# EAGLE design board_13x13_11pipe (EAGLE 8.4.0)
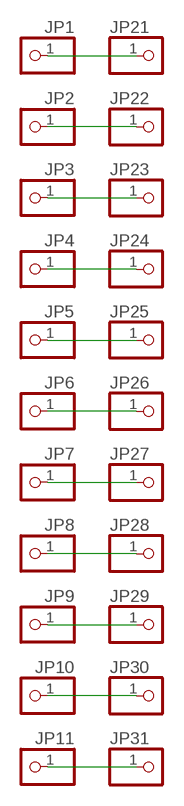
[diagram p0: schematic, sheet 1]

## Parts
JP1  PINHD-1X1CB  [1X01-CLEANBIG]
JP2  PINHD-1X1CB  [1X01-CLEANBIG]
JP3  PINHD-1X1CB  [1X01-CLEANBIG]
JP4  PINHD-1X1CB  [1X01-CLEANBIG]
JP5  PINHD-1X1CB  [1X01-CLEANBIG]
JP6  PINHD-1X1CB  [1X01-CLEANBIG]
JP7  PINHD-1X1CB  [1X01-CLEANBIG]
JP8  PINHD-1X1CB  [1X01-CLEANBIG]
JP9  PINHD-1X1CB  [1X01-CLEANBIG]
JP10  PINHD-1X1CB  [1X01-CLEANBIG]
JP11  PINHD-1X1CB  [1X01-CLEANBIG]
JP21  PINHD-1X1CB  [1X01-CLEANBIG]
JP22  PINHD-1X1CB  [1X01-CLEANBIG]
JP23  PINHD-1X1CB  [1X01-CLEANBIG]
JP24  PINHD-1X1CB  [1X01-CLEANBIG]
JP25  PINHD-1X1CB  [1X01-CLEANBIG]
JP26  PINHD-1X1CB  [1X01-CLEANBIG]
JP27  PINHD-1X1CB  [1X01-CLEANBIG]
JP28  PINHD-1X1CB  [1X01-CLEANBIG]
JP29  PINHD-1X1CB  [1X01-CLEANBIG]
JP30  PINHD-1X1CB  [1X01-CLEANBIG]
JP31  PINHD-1X1CB  [1X01-CLEANBIG]

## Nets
N$1: JP1.1 JP21.1
N$2: JP2.1 JP22.1
N$3: JP3.1 JP23.1
N$4: JP4.1 JP24.1
N$5: JP5.1 JP25.1
N$6: JP6.1 JP26.1
N$7: JP7.1 JP27.1
N$8: JP8.1 JP28.1
N$9: JP9.1 JP29.1
N$10: JP10.1 JP30.1
N$11: JP11.1 JP31.1

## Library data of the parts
JP1-JP11 JP21-JP31 = adafruit:PINHD-1X1: Pin header 1x1 for 0.1" spacing

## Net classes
0 default: width 3.048 mm, drill 0.762 mm, clearance 1.524 mm

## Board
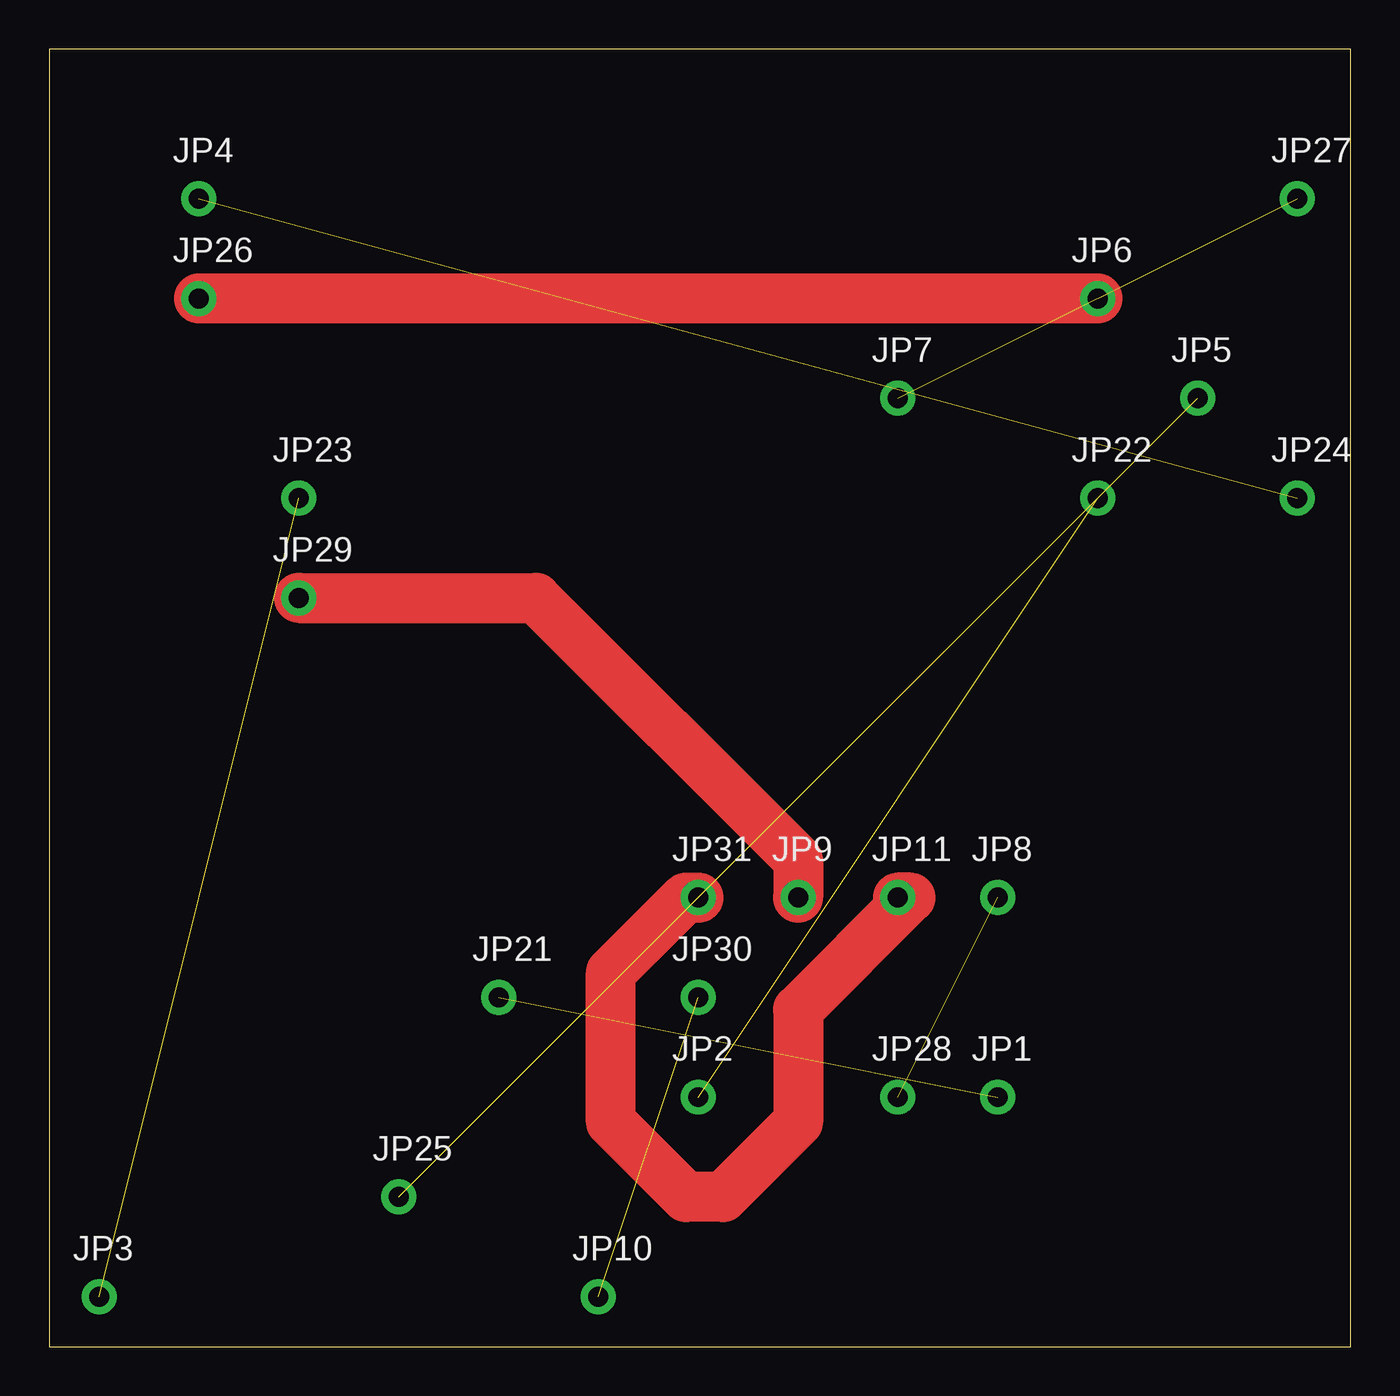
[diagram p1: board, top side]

Size 66.22 x 66.03 mm. Coordinates in mm from the lower left corner, seen from the top.
Outline: 0,0 66.22,0 66.22,66.03 0,66.03 0,0
Copper layers (1*16): Top 0.035mm / dielectric 1.5mm / Bottom 0.035mm
Design rules "default": minimum track width 6mil, minimum drill 0.35mm, track to track 6mil, track to pad 6mil, pad to pad 6mil, via to via 6mil, smd to smd 6mil, copper to edge 40mil, drill to drill 6mil, minimum pad ring 10mil, minimum via ring 8mil, stop-mask expansion 4mil, vias tented up to drill 0mil, thermal gap 10mil

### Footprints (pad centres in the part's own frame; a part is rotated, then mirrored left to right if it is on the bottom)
1X01-CLEANBIG = drill 1.016 pad 1.778: 1 0,0

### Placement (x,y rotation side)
JP1  48.26,12.7 0 top
JP2  33.02,12.7 0 top
JP3  2.54,2.54 0 top
JP4  7.62,58.42 0 top
JP5  58.42,48.26 0 top
JP6  53.34,53.34 0 top
JP7  43.18,48.26 0 top
JP8  48.26,22.86 0 top
JP9  38.1,22.86 0 top
JP10  27.94,2.54 0 top
JP11  43.18,22.86 0 top
JP21  22.86,17.78 0 top
JP22  53.34,43.18 0 top
JP23  12.7,43.18 0 top
JP24  63.5,43.18 0 top
JP25  17.78,7.62 0 top
JP26  7.62,53.34 0 top
JP27  63.5,58.42 0 top
JP28  43.18,12.7 0 top
JP29  12.7,38.1 0 top
JP30  33.02,17.78 0 top
JP31  33.02,22.86 0 top

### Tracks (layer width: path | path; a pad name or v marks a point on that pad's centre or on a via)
N$1  (1 unrouted)
N$2  (1 unrouted)
N$3  (1 unrouted)
N$4  (1 unrouted)
N$5  (1 unrouted)
N$6
  Top 2.54: JP6.1 JP26.1
N$7  (1 unrouted)
N$8  (1 unrouted)
N$9
  Top 2.54: JP9.1 38.1,24.77 24.77,38.1 JP29.1
N$10  (1 unrouted)
N$11
  Top 2.54: JP31.1 32.38,22.86 28.57,19.05 28.57,11.43 32.38,7.62 34.29,7.62 38.1,11.43 38.1,17.14 43.81,22.86 JP11.1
